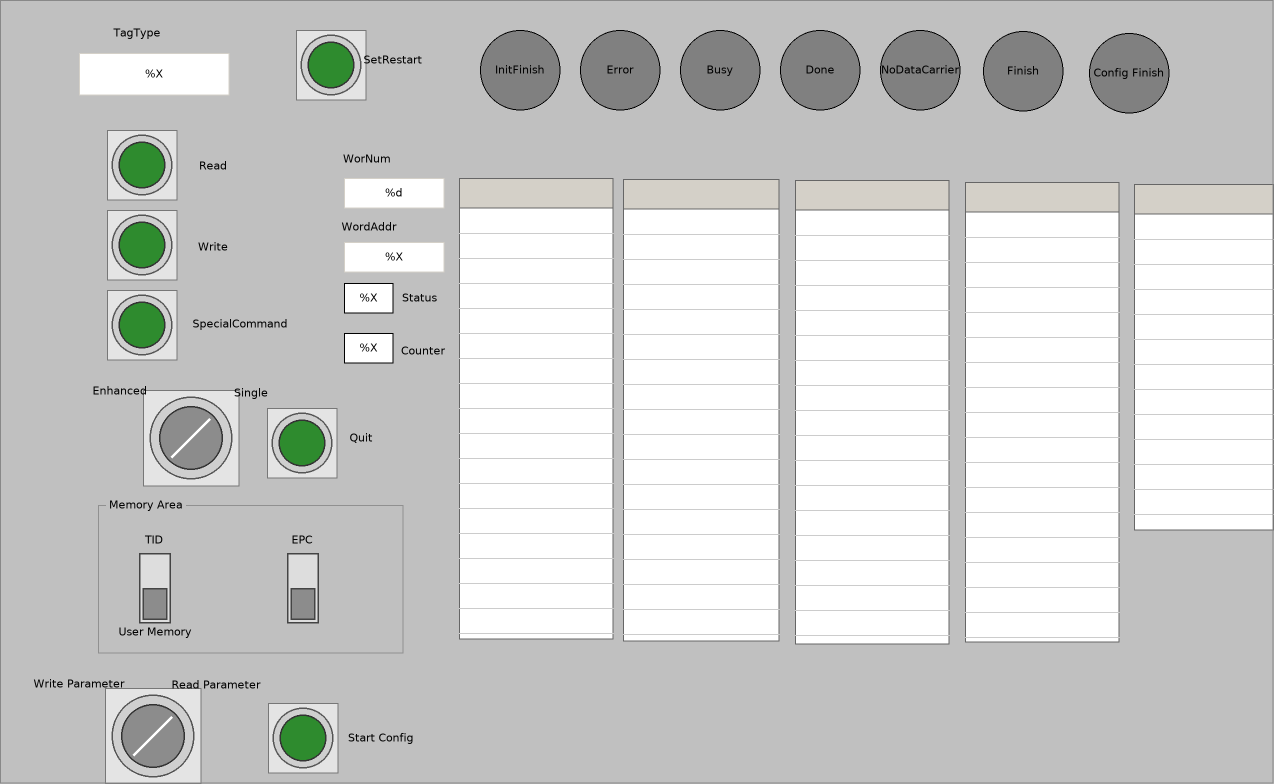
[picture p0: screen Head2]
VISUALIZATION Head2  // 1274x784
    GroupBox (98,497 305x156), "Memory Area"
        DipSwitch (22,56 70x70), variable: MAIN.Head2UserMemoryUID, behaviour: TOGGLE, style: Switch-DipSwitch-Gray
        DipSwitch (170,56 70x70), variable: MAIN.Head2EPC, behaviour: TOGGLE, style: Switch-DipSwitch-Gray
        Label (129,28 150x30), "EPC"
    PushSwitch (107,130 70x70), variable: MAIN.Head2Read, behaviour: TAP, style: Switch-PushSwitch-Green
    PushSwitch (107,210 70x70), variable: MAIN.Head2Write, behaviour: TAP, style: Switch-PushSwitch-Green
    RotarySwitch (138,390 106x96), variable: MAIN.Head2SingleEnhanced, behaviour: TOGGLE, style: Switch-RotarySwitch-Gray
    Textfield (79,53 150x42), "%X", tooltip "TagType", text variable: MAIN.Head2TagType
        OnMouseDown: write MAIN.Head2TagType via Default
    Table (459,178 154x461), data array: MAIN.IC_KP2_2HB21_IQH3_SF_Head2.IDENTControl_FB_SF.INDATA
        p1892666644: MAIN.Data_Channel.InData[2][INDEX]
        p3854506369: MAIN.IC_KP2_2HB21_IQH3_SF_Head2.IDENTControl_FB_SF.INDATA[INDEX]
    Table (623,179 156x462), data array: MAIN.IC_KP2_2HB21_IQH3_SF_Head2.IDENTControl_FB_SF.OUTDATA
        p1892666644: MAIN.Data_Channel.OutData[2][INDEX]
        p3854506369: MAIN.IC_KP2_2HB21_IQH3_SF_Head2.IDENTControl_FB_SF.OUTDATA[INDEX]
    Textfield (344,242 100x30), "%X", text variable: MAIN.Head1StartAddress
        OnMouseClick: write MAIN.Head2StartAddress via Default
    Textfield (344,178 100x30), "%d", text variable: MAIN.Head1WordNum
        OnMouseClick: write MAIN.Head2WordNum via Default
    PushSwitch (296,30 70x70), variable: MAIN.Head2SetRestart, behaviour: TAP, style: Switch-PushSwitch-Green
    PushSwitch (267,408 70x70), tooltip "Cancel "Enhanced"-Command", variable: MAIN.Head2Quit, behaviour: TAP, style: Switch-PushSwitch-Green
    PushSwitch (107,290 70x70), variable: MAIN.Head2SpecialCommand, behaviour: TAP, style: Switch-PushSwitch-Green
    Table (1134,184 140x346), data array: MAIN.Head2Data.SpecialCommand
        p1892666644: MAIN.Data_Channel.SpecialCommand[2][INDEX]
        p3854506369: MAIN.Head2Data.SpecialCommand[INDEX]
        Columns.Column.[0].Template: OnMouseDown: write the text variable via Default
    Rectangle (344,283 49x30), "%X", text variable: MAIN.Head2Status, input disabled if: TRUE
    Rectangle (344,333 49x30), "%X", text variable: MAIN.Head2ReplyCounter, input disabled if: TRUE
    Ellipse (480,30 80x80), "InitFinish", colour toggle: MAIN.Head2InitFinish
    Ellipse (580,30 80x80), "Error", colour toggle: MAIN.Head2Error
    Ellipse (680,30 80x80), "Busy", colour toggle: MAIN.Head2Busy
    Ellipse (780,30 80x80), "Done", colour toggle: MAIN.Head2Done
    Ellipse (880,30 80x80), "NoDataCarrier", colour toggle: MAIN.Head2NoDataCarrier
    Label (62,18 150x30), "TagType"
    Label (292,144 150x30), "WorNum"
    Label (294,212 150x30), "WordAddr"
    Label (346,283 147x30), "Status"
    Label (346,336 154x30), "Counter"
    Label (138,151 150x30), "Read"
    Label (138,232 150x30), "Write"
    Label (165,309 150x30), "SpecialCommand"
    Label (45,376 150x30), "Enhanced"
    Label (176,378 150x30), "Single"
    Label (286,423 150x30), "Quit"
    Label (79,525 150x30), "TID"
    Label (80,617 150x30), "User Memory"
    Ellipse (983,31 80x80), "Finish", colour toggle: MAIN.Head2Finish
    Table (795,180 154x464), data array: MAIN.Head2Data.ReadData
        p1892666644: MAIN.Data_Channel.SpecialCommand[2][INDEX]
        p3854506369: MAIN.Head2Data.ReadData[INDEX]
        Columns.Column.[0].Template: OnMouseDown: write the text variable via Default
    Table (965,182 154x460), data array: MAIN.Head2Data.WriteData
        p1892666644: MAIN.Data_Channel.SpecialCommand[2][INDEX]
        p3854506369: MAIN.Head2Data.WriteData[INDEX]
        Columns.Column.[0].Template: OnMouseDown: write the text variable via Default
    Label (318,45 150x30), "SetRestart"
    RotarySwitch (100,688 106x96), variable: MAIN.Head1WriteParameter, behaviour: TOGGLE, style: Switch-RotarySwitch-Gray
    Label (141,670 150x30), "Read Parameter"
    Label (4,669 150x30), "Write Parameter"
    PushSwitch (268,703 70x70), variable: MAIN.Head2StartConfig, behaviour: TAP, style: Switch-PushSwitch-Green
    Label (306,724 150x28), "Start Config"
    Ellipse (1089,33 80x80), "Config Finish", colour toggle: MAIN.Head2EndConfig
END_VISUALIZATION
